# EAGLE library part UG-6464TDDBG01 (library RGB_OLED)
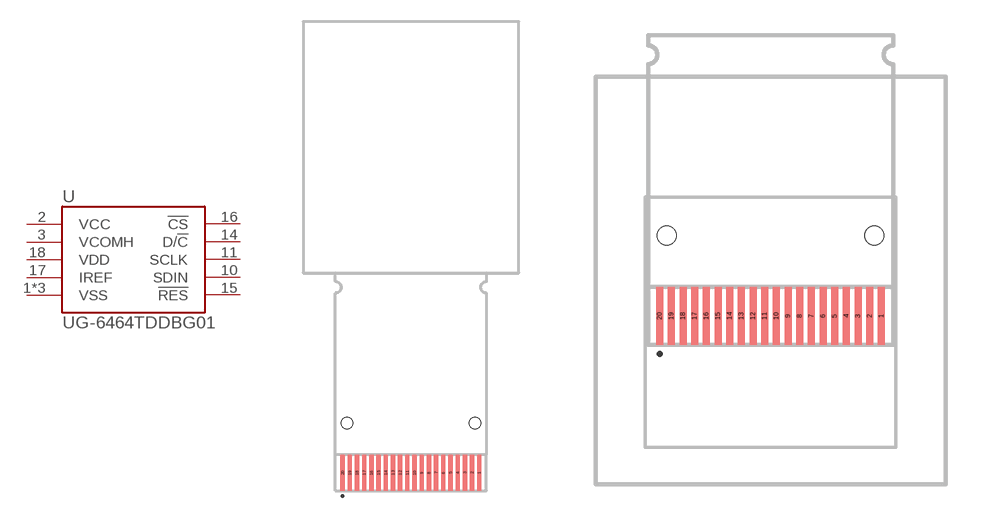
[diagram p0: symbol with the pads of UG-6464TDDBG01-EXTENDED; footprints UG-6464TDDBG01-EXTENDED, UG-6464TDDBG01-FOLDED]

Designator prefix U

## UG-6464TDDBG01-EXT  [UG-6464TDDBG01-EXTENDED]
1  VSS
2  VCC
3  VCOMH
10  SDIN
11  SCLK
14  D/!C
15  !RES
16  !CS
17  IREF
18  VDD
19  VSS
20  VSS

## UG-6464TDDBG01-FLD  [UG-6464TDDBG01-FOLDED]
Pads as for UG-6464TDDBG01-EXTENDED

## Footprint UG-6464TDDBG01-EXTENDED (pad centres in mm)
smd 0.3 x 2.5: 1 4.75,1.25; 2 4.25,1.25; 3 3.75,1.25; 4 3.25,1.25; 5 2.75,1.25; 6 2.25,1.25; 7 1.75,1.25; 8 1.25,1.25; 9 0.75,1.25; 10 0.25,1.25; 11 -0.25,1.25; 12 -0.75,1.25; 13 -1.25,1.25; 14 -1.75,1.25; 15 -2.25,1.25; 16 -2.75,1.25; 17 -3.25,1.25; 18 -3.75,1.25; 19 -4.25,1.25; 20 -4.75,1.25
hole 0.8 at -4.45,4.7
hole 0.8 at 4.45,4.7

## Footprint UG-6464TDDBG01-FOLDED (pad centres in mm)
smd 0.3 x 2.5: 1 4.75,1.25; 2 4.25,1.25; 3 3.75,1.25; 4 3.25,1.25; 5 2.75,1.25; 6 2.25,1.25; 7 1.75,1.25; 8 1.25,1.25; 9 0.75,1.25; 10 0.25,1.25; 11 -0.25,1.25; 12 -0.75,1.25; 13 -1.25,1.25; 14 -1.75,1.25; 15 -2.25,1.25; 16 -2.75,1.25; 17 -3.25,1.25; 18 -3.75,1.25; 19 -4.25,1.25; 20 -4.75,1.25
hole 0.8 at -4.45,4.7
hole 0.8 at 4.45,4.7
